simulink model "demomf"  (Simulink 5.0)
settings: Solver=ode45  StartTime=0.0  StopTime=200  FixedStep=0.1  RelTol=1e-3
libraries: simulink_extras x2, MarineGNC x1, simulink x1

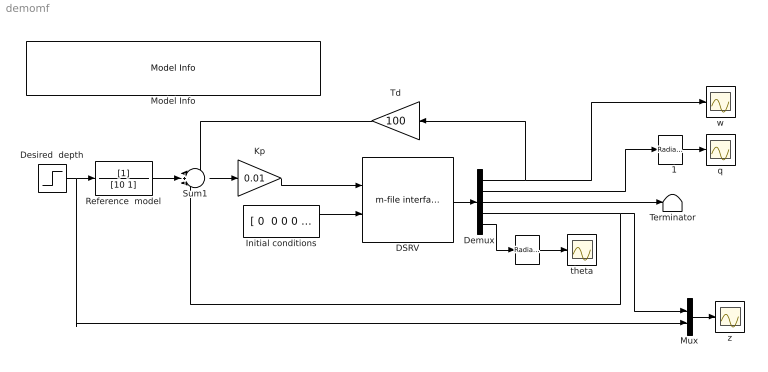
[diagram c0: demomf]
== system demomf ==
  "   " : simulink_extras/Transformations/Radians to Degrees
  "   1" : simulink_extras/Transformations/Radians to Degrees
  DSRV : MarineGNC/Models/Vessels/m-file interface  vessmodel='DSRV'  dimu_model=1  dimx_model=5
  Demux : Demux  Outputs=5
  Desired  depth : Step  Time=30  After=50  SampleTime=0
  Initial conditions : Constant  Value="[ 0  0 0 0 0]"
  Kp : Gain  Gain=0.01
  Model Info : simulink/Model-Wide Utilities/Model Info  InitialBlockCM=None  BlockCM=None  Frame=on  DisplayStringWithTags=|  HorizontalTextAlignment=Left  LeftAlignmentValue=0.02  SourceBlockDiagram=demomf  TagMaxNumber=20
      | Deep submergence rescue vehicle (DSRV) depth control system
      | Simulink interface to the GNC Toolbox m-file vessel models
      | %<Creator>Author: Thor I. Fossen
      | %<LastModificationDate>
  Mux : Mux  Inputs=2
  Reference  model : TransferFcn  Denominator=[10 1]
  Sum1 : Sum  Inputs=-+-
  Td : Gain  Orientation=left  Gain=100
  Terminator : Terminator
  q : Scope
  theta : Scope
  w : Scope
  z : Scope
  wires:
  Initial conditions/1 -> DSRV/2
  DSRV/1 -> Demux/1
  Demux/1 -> w/1, Td/1
  Demux/2 -> "   1"/1
  Kp/1 -> DSRV/1
  Desired  depth/1 -> Reference  model/1, Mux/2
  Reference  model/1 -> Sum1/2
  Sum1/1 -> Kp/1
  Td/1 -> Sum1/1
  "   "/1 -> theta/1
  "   1"/1 -> q/1
  Mux/1 -> z/1
  Demux/4 -> Sum1/3, Mux/1
  Demux/3 -> Terminator/1
  Demux/5 -> "   "/1
